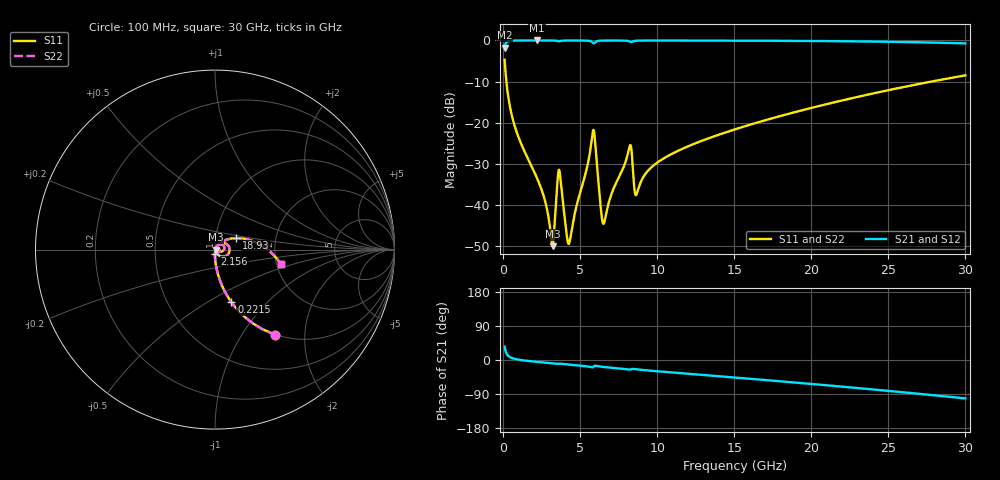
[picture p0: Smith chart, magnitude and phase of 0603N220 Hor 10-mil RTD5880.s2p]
# GHz S MA R 50
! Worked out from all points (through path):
!   3201 points, 100 MHz to 30 GHz, reference 50 ohm
!   highest |S21| = -0.01 dB at 2.202 GHz (marker M1); lowest = -1.8 dB at 100 MHz (marker M2)
!   group delay of S21, straight-line fit = 9.56 ps
!   lowest |S11| = -50.0 dB at 3.211 GHz (marker M3), VSWR 1.01, Z = 50.3 - j0.127 ohm
!   |S11| at or under -10 dB: 214.3 MHz to 27.81 GHz (27.59 GHz wide, 197 % of centre)
!   |S22| runs from -50.0 to -4.7 dB; largest |S21 - S12| = 0
!   S11 on the Smith chart (normalised r, x): 100 MHz: 0.99, -1.43; 221.5 MHz: 0.99, -0.64; 2.156 GHz: 1.00, -0.04; 18.93 GHz: 1.25, +0.16; 30 GHz: 2.11, -0.39
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0.1  0.5822 -54.6  0.8127 35.3  0.8127 35.3  0.5822 -54.6
0.2214687  0.3069 -72.7  0.9513 17.2  0.9513 17.2  0.3069 -72.7
0.7914375  0.08638 -86.7  0.9954 2.7  0.9954 2.7  0.08638 -86.7
2.155625  0.02213 -91.3  0.9984 -4.8  0.9984 -4.8  0.02213 -91.3
2.202344  0.02114 -91.2  0.9984 -5.0  0.9984 -5.0  0.02114 -91.2
2.71625  0.01131 -88.4  0.9982 -7.0  0.9982 -7.0  0.01131 -88.4
3.211469  0.003147 -23.7  0.9969 -9.0  0.9969 -9.0  0.003147 -23.7
3.622594  0.02672 -13.7  0.9733 -10.1  0.9733 -10.1  0.02672 -13.7
4.257969  0.003346 -3.9  0.9966 -12.0  0.9966 -12.0  0.003346 -3.9
5.089563  0.0161 61.4  0.9961 -15.2  0.9961 -15.2  0.0161 61.4
5.837063  0.07958 10.4  0.9296 -18.6  0.9296 -18.6  0.07958 10.4
5.986562  0.05433 -46.0  0.9529 -15.2  0.9529 -15.2  0.05433 -46.0
6.369656  0.0081 -42.5  0.9926 -17.7  0.9926 -17.7  0.0081 -42.5
6.5285  0.005916 2.8  0.9944 -18.4  0.9944 -18.4  0.005916 2.8
8.191688  0.04982 32.9  0.9727 -25.3  0.9727 -25.3  0.04982 32.9
8.649531  0.01335 24.2  0.9911 -24.7  0.9911 -24.7  0.01335 24.2
10.06978  0.0333 54.1  0.9959 -30.0  0.9959 -30.0  0.0333 54.1
15.05  0.0829 41.1  0.9925 -46.3  0.9925 -46.3  0.0829 41.1
18.92766  0.1341 28.7  0.9862 -59.4  0.9862 -59.4  0.1341 28.7
20.03956  0.1516 24.9  0.9835 -63.3  0.9835 -63.3  0.1516 24.9
25.01978  0.2486 7.2  0.9626 -81.5  0.9626 -81.5  0.2486 7.2
30  0.3757 -12.3  0.9196 -101.3  0.9196 -101.3  0.3757 -12.3
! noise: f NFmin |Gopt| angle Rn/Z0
0.1  0.0003033  0.9214  0.4195  0.000853
3.417  0.007301  0.8903  9.606  0.01438
6.743  0.008074  0.8131  18.89  0.008778
10.06  0.008658  0.7508  27.97  0.006602
13.39  0.01026  0.7267  36.88  0.006736
16.7  0.0122  0.718  45.57  0.007307
20.03  0.01423  0.7145  54.05  0.007863
23.35  0.01636  0.7145  62.26  0.008375
26.67  0.01865  0.7175  70.25  0.008848
30  0.02113  0.7227  77.99  0.009283
